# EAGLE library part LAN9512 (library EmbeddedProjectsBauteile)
USB 2.0 Hub and 10/100 Ethernet Controller
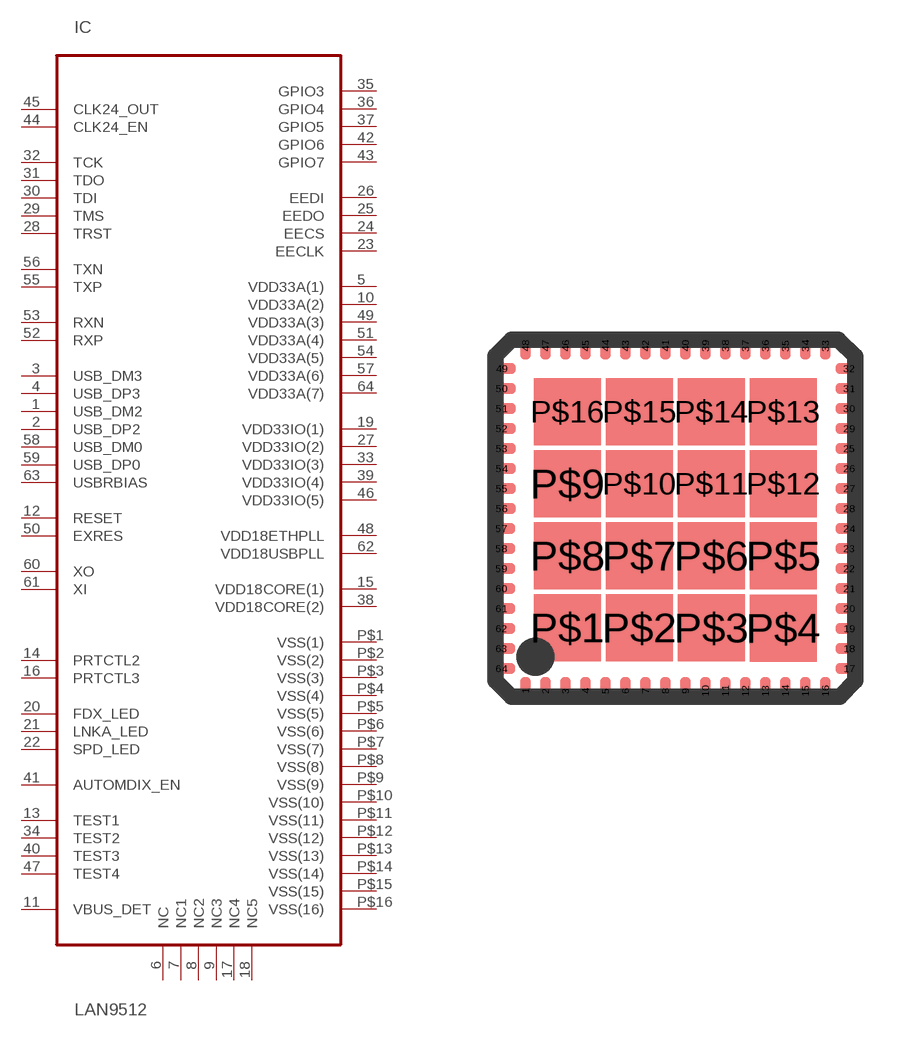
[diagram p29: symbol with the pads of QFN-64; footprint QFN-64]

Designator prefix IC

## LAN9512 (EP: 401099)  [QFN-64]
1  USB_DM2
2  USB_DP2
3  USB_DM3
4  USB_DP3
5  VDD33A(1)  pwr
6  NC  nc
7  NC1  nc
8  NC2  nc
9  NC3  nc
10  VDD33A(2)  pwr
11  VBUS_DET  in
12  RESET  in
13  TEST1
14  PRTCTL2
15  VDD18CORE(1)  pwr
16  PRTCTL3
17  NC4  nc
18  NC5  nc
19  VDD33IO(1)  pwr
20  FDX_LED
21  LNKA_LED
22  SPD_LED
23  EECLK
24  EECS  out
25  EEDO  out
26  EEDI  in
27  VDD33IO(2)  pwr
28  TRST  in
29  TMS  in
30  TDI  in
31  TDO
32  TCK  out
33  VDD33IO(3)  pwr
34  TEST2
35  GPIO3
36  GPIO4
37  GPIO5
38  VDD18CORE(2)  pwr
39  VDD33IO(4)
40  TEST3
41  AUTOMDIX_EN
42  GPIO6
43  GPIO7
44  CLK24_EN  in
45  CLK24_OUT
46  VDD33IO(5)
47  TEST4
48  VDD18ETHPLL  pwr
49  VDD33A(3)  pwr
50  EXRES  in
51  VDD33A(4)  pwr
52  RXP
53  RXN
54  VDD33A(5)  pwr
55  TXP
56  TXN
57  VDD33A(6)  pwr
58  USB_DM0
59  USB_DP0
60  XO  out
61  XI  in
62  VDD18USBPLL
63  USBRBIAS  in
64  VDD33A(7)  pwr
P$1  VSS(1)  pwr
P$2  VSS(2)  pwr
P$3  VSS(3)  pwr
P$4  VSS(4)  pwr
P$5  VSS(5)  pwr
P$6  VSS(6)  pwr
P$7  VSS(7)  pwr
P$8  VSS(8)  pwr
P$9  VSS(9)  pwr
P$10  VSS(10)  pwr
P$11  VSS(11)  pwr
P$12  VSS(12)  pwr
P$13  VSS(13)  pwr
P$14  VSS(14)  pwr
P$15  VSS(15)  pwr
P$16  VSS(16)  pwr

## Footprint QFN-64 (pad centres in mm)
smd 0.27 x 0.7: 1 0.98,0.42; 2 1.48,0.42; 3 1.98,0.42; 4 2.48,0.42; 5 2.98,0.42; 6 3.48,0.42; 7 3.98,0.42; 8 4.48,0.42; 9 4.98,0.42; 10 5.48,0.42; 11 5.98,0.42; 12 6.48,0.42; 13 6.98,0.42; 14 7.48,0.42; 15 7.98,0.42; 16 8.48,0.42; 33 8.48,9.05; 34 7.98,9.05; 35 7.48,9.05; 36 6.98,9.05; 37 6.48,9.05; 38 5.98,9.05; 39 5.48,9.05; 40 4.98,9.05; 41 4.48,9.05; 42 3.98,9.05; 43 3.48,9.05; 44 2.98,9.05; 45 2.48,9.05; 46 1.98,9.05; 47 1.48,9.05; 48 0.98,9.05
smd 0.7 x 0.27: 17 9.08,0.98; 18 9.08,1.48; 19 9.08,1.98; 20 9.08,2.48; 21 9.08,2.98; 22 9.08,3.48; 23 9.08,3.98; 24 9.08,4.48; 25 9.08,6.48; 26 9.08,5.98; 27 9.08,5.48; 28 9.08,4.98; 29 9.08,6.98; 30 9.08,7.48; 31 9.08,7.98; 32 9.08,8.48; 49 0.39,8.48; 50 0.39,7.98; 51 0.39,7.48; 52 0.39,6.98; 53 0.39,6.48; 54 0.39,5.98; 55 0.39,5.48; 56 0.39,4.98; 57 0.38,4.48; 58 0.38,3.98; 59 0.38,3.48; 60 0.38,2.98; 61 0.38,2.48; 62 0.38,1.98; 63 0.38,1.48; 64 0.38,0.98
smd 1.676 x 1.676: P$1 2.03,2; P$2 3.83,2; P$3 5.63,2; P$4 7.43,1.99; P$5 7.43,3.8; P$6 5.63,3.8; P$7 3.83,3.8; P$8 2.03,3.8; P$9 2.03,5.6; P$10 3.83,5.6; P$11 5.63,5.6; P$12 7.43,5.6; P$13 7.43,7.4; P$14 5.63,7.4; P$15 3.83,7.4; P$16 2.03,7.4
